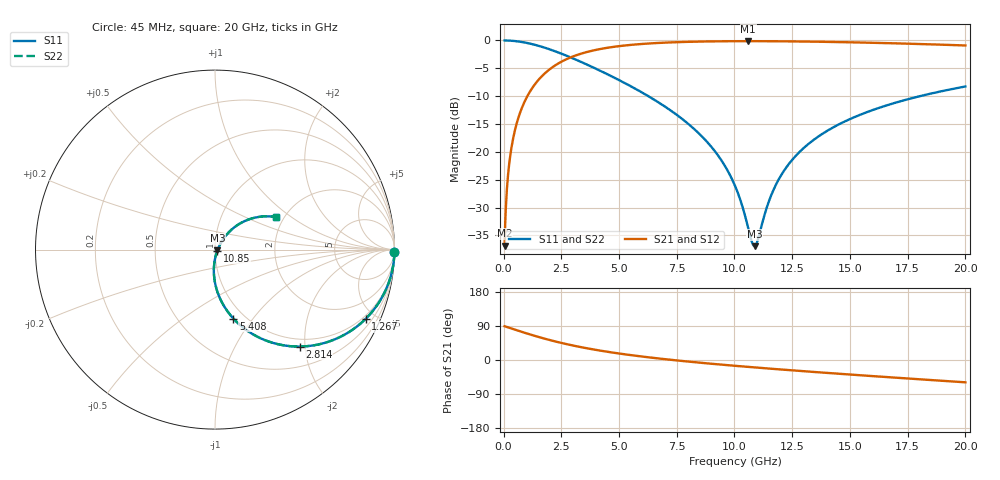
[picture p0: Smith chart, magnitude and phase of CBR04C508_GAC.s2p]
! S-parameter model data by Modelithics Inc.  support@modelithics.com 813-866-6335  Tampa FL USA
! S-Parameter data specifications:
! Substrate: 20-mil Rogers 4350B, substrate thickness, H=0.508mm, Dielectric constant, Er=3.75
! PCB Mounting Pad Footprint: Pad width, PadW=0.52mm , Pad length, PadL=0.52mm , Pad gap, PadG (edge-to-edge)=0.28mm , Reference planes=1.32mm apart
#  GHz  S  MA  R 50
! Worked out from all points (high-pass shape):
!   801 points, 45 MHz to 20 GHz, reference 50 ohm
!   highest |S21| = -0.13 dB at 10.6 GHz (marker M1); lowest = -36.8 dB at 45 MHz (marker M2)
!   |S21| within 3 dB of the highest: 2.853 GHz to end of sweep
!   lowest |S11| = -36.9 dB at 10.87 GHz (marker M3), VSWR 1.03, Z = 51.4 - j0.495 ohm
!   |S11| at or under -10 dB: 6.269 GHz to 18.03 GHz (11.76 GHz wide, 96.8 % of centre)
!   |S22| runs from -36.9 to 0.0 dB; largest |S21 - S12| = 0
!   S11 on the Smith chart (normalised r, x): 45 MHz: open; 1.267 GHz: 0.84, -4.42; 2.814 GHz: 0.85, -1.89; 5.408 GHz: 0.88, -0.81; 10.85 GHz: 1.03, -0.01; 20 GHz: 1.82, +0.78
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0.045  0.9999 -0.9  0.01445 89.1  0.01445 89.1  0.9999 -0.9
0.219606  0.9975 -4.4  0.07038 85.6  0.07038 85.6  0.9975 -4.4
0.419156  0.991 -8.4  0.1336 81.5  0.1336 81.5  0.991 -8.4
0.768369  0.9704 -15.3  0.2406 74.6  0.2406 74.6  0.9704 -15.3
1.267244  0.9238 -24.7  0.3809 65.2  0.3809 65.2  0.9238 -24.7
1.990612  0.8329 -37.0  0.55 52.8  0.55 52.8  0.8329 -37.0
2.813756  0.717 -48.9  0.6921 40.7  0.6921 40.7  0.717 -48.9
3.387462  0.6375 -56.0  0.7644 33.5  0.7644 33.5  0.6375 -56.0
5.407906  0.3983 -75.0  0.9082 13.7  0.9082 13.7  0.3983 -75.0
6.704981  0.2785 -83.8  0.9498 4.1  0.9498 4.1  0.2785 -83.8
8.775313  0.1254 -92.9  0.9794 -8.6  0.9794 -8.6  0.1254 -92.9
9.473738  0.08156 -93.2  0.9833 -12.5  0.9833 -12.5  0.08156 -93.2
10.0225  0.04962 -89.5  0.985 -15.3  0.985 -15.3  0.04962 -89.5
10.59621  0.02062 -65.3  0.9855 -18.2  0.9855 -18.2  0.02062 -65.3
10.84564  0.0143 -25.1  0.9854 -19.5  0.9854 -19.5  0.0143 -25.1
10.87059  0.01425 -19.7  0.9854 -19.6  0.9854 -19.6  0.01425 -19.7
11.02025  0.01647 8.9  0.9852 -20.3  0.9852 -20.3  0.01647 8.9
11.51913  0.03737 44.0  0.9843 -22.7  0.9843 -22.7  0.03737 44.0
11.91822  0.05674 50.0  0.983 -24.6  0.983 -24.6  0.05674 50.0
13.36496  0.1253 51.4  0.9757 -31.2  0.9757 -31.2  0.1253 51.4
16.68248  0.2651 40.6  0.9455 -45.4  0.9455 -45.4  0.2651 40.6
20  0.3863 28.1  0.9015 -58.9  0.9015 -58.9  0.3863 28.1
